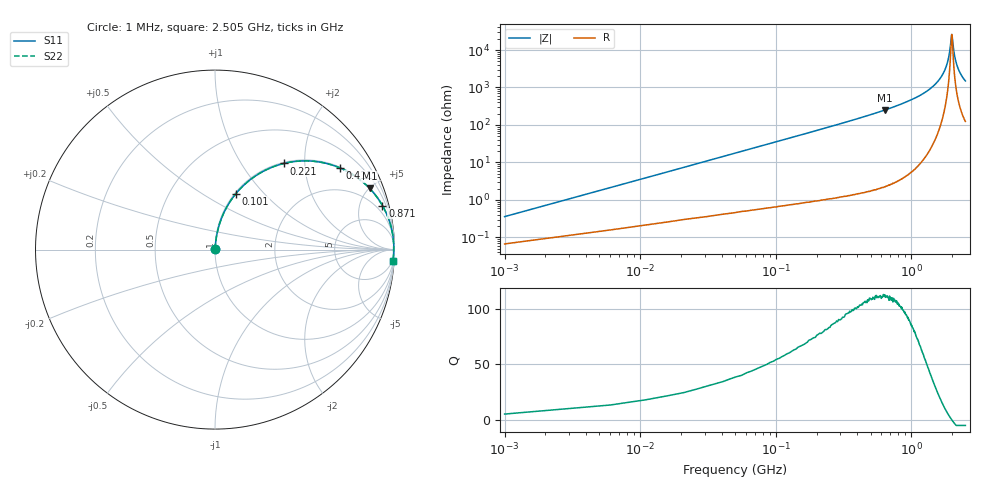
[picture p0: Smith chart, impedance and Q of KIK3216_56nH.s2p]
!version-2
!date-01.2022
!Series
# MHz S RI R 50
!Freq ReS11 ImS11 ReS21 ImS21 ReS12 ImS12 ReS22 ImS22
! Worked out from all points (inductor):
!   501 points, 1 MHz to 2.505 GHz, reference 50 ohm
!   read as one part in series: L = 56 nH near 11 MHz
!   highest Q = 112 at 641 MHz (marker M1), where L = 62.5 nH
!   self-resonance near 1.985 GHz
!   S11 on the Smith chart (normalised r, x): 1 MHz: 1.00, +0.01; 101 MHz: 1.01, +0.71; 221 MHz: 1.02, +1.57; 411 MHz: 1.03, +3.02; 871 MHz: 1.08, +7.59; 2.505 GHz: 3, -30
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1  0.000662 0.00351  0.9993 -0.00351  0.9993 -0.00351  0.000662 0.00351
16  0.00573 0.0558  0.9943 -0.0558  0.9943 -0.0558  0.00573 0.0558
31  0.0152 0.1071  0.9848 -0.1071  0.9848 -0.1071  0.0152 0.1071
61  0.0485 0.2034  0.9515 -0.2034  0.9515 -0.2034  0.0485 0.2034
101  0.1171 0.3125  0.8829 -0.3125  0.8829 -0.3125  0.1171 0.3125
221  0.3842 0.4801  0.6158 -0.4801  0.6158 -0.4801  0.3842 0.4801
411  0.6937 0.4561  0.3063 -0.4561  0.3063 -0.4561  0.6937 0.4561
421  0.7046 0.4514  0.2954 -0.4514  0.2954 -0.4514  0.7046 0.4514
641  0.8616 0.3409  0.1384 -0.3409  0.1384 -0.3409  0.8616 0.3409
836  0.9253 0.258  0.0747 -0.258  0.0747 -0.258  0.9253 0.258
871  0.9329 0.2451  0.067 -0.2451  0.067 -0.2451  0.9329 0.2451
1255  0.9793 0.1337  0.0207 -0.1337  0.0207 -0.1337  0.9793 0.1337
1675  0.9945 0.0491  0.00548 -0.0491  0.00548 -0.0491  0.9945 0.0491
1785  0.9957 0.0308  0.00426 -0.0308  0.00426 -0.0308  0.9957 0.0308
1865  0.9962 0.0183  0.00383 -0.0183  0.00383 -0.0183  0.9962 0.0183
1920  0.9963 0.01  0.00374 -0.01  0.00374 -0.01  0.9963 0.01
1985  0.9962 0.000516  0.00381 -0.000516  0.00381 -0.000516  0.9962 0.000516
2000  0.9961 -0.00163  0.00386 0.00163  0.00386 0.00163  0.9961 -0.00163
2050  0.9959 -0.00865  0.00408 0.00865  0.00408 0.00865  0.9959 -0.00865
2090  0.9957 -0.0141  0.00432 0.0141  0.00432 0.0141  0.9957 -0.0141
2245  0.9942 -0.0345  0.00581 0.0345  0.00581 0.0345  0.9942 -0.0345
2505  0.9901 -0.0656  0.00989 0.0656  0.00989 0.0656  0.9901 -0.0656
